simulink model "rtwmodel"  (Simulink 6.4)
settings: Solver=ode4  StartTime=0.0  StopTime=10.0  FixedStep=.0242  RelTol=1e-3
libraries: ballbeam x1

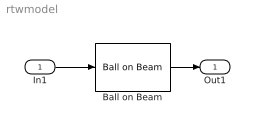
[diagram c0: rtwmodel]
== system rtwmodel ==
  In1 : Inport
  Ball on Beam : ballbeam/Ball on Beam  SystemSampleTime=-1
  Out1 : Outport
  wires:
  Ball on Beam/1 -> Out1/1
  In1/1 -> Ball on Beam/1
